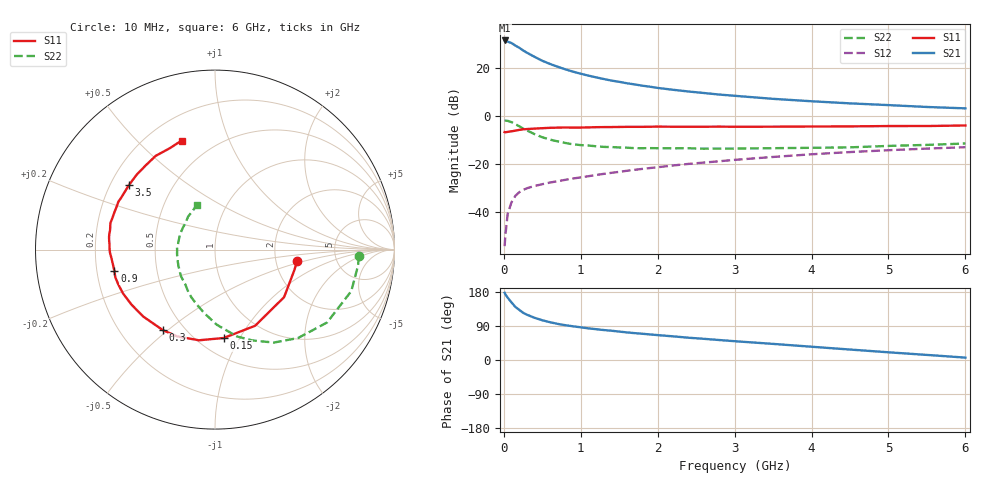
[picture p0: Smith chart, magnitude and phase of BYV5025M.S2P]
! SIEMENS Small Signal Semiconductors
! BFY420
! Si NPN RF SIEGET Grounded Emitter Transistor in MICRO-X
! VCE = 0.5 V  IC = 25 mA
! Common Emitter S-Parameters:  October  1996
# GHz  S  MA  R  50
!  f  S11  S21  S12  S22
! GHz  MAG  ANG  MAG  ANG  MAG  ANG  MAG  ANG
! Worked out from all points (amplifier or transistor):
!   36 points, 10 MHz to 6 GHz, reference 50 ohm
!   highest |S21| = 31.6 dB at 10 MHz (marker M1)
!   |S21| within 3 dB of that: start of sweep to 197 MHz
!   unconditionally stable (mu >= 1): start of sweep to 23.53 MHz; 1.099 GHz to end of sweep
!   at 250 MHz: K = 0.42, MSG = 29.2 dB, |S12| = -30.9 dB
!   at 1.4 GHz: K = 1.08, MAG = 17.6 dB, |S12| = -23.7 dB
!   at 6 GHz: K = 1.18, MAG = 5.6 dB, |S12| = -13.0 dB
!   S11 on the Smith chart (normalised r, x): 10 MHz: 2.64, -0.43; 150 MHz: 0.66, -0.86; 300 MHz: 0.38, -0.48; 900 MHz: 0.27, -0.10; 3.5 GHz: 0.28, +0.31; 6 GHz: 0.34, +0.68
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0.01  0.4621 -7.9  38.1 177.4  0.0019 97.3  0.8015 -2.6
0.02  0.4564 -14.8  37.83 173.2  0.0032 85.3  0.8022 -6.2
0.05  0.4673 -34.5  36.03 164.4  0.009 79.1  0.7939 -16.9
0.1  0.4796 -62.2  33.61 151.9  0.0158 69.6  0.745 -33.0
0.15  0.4949 -84.4  29.78 140.1  0.0215 60.8  0.6758 -46.8
0.2  0.5132 -100.1  26.81 132.4  0.0255 56.7  0.6128 -57.7
0.25  0.5273 -113.5  23.61 124.7  0.0285 51.8  0.5469 -67.7
0.3  0.5345 -122.9  21.12 119.5  0.0309 49.4  0.4992 -75.8
0.4  0.5466 -136.9  17.29 111.3  0.0345 47.5  0.4183 -88.7
0.5  0.5571 -146.6  14.32 104.9  0.0376 46.7  0.3602 -99.3
0.6  0.5674 -154.3  12.29 99.7  0.0407 46.1  0.3215 -108.6
0.7  0.5724 -159.9  10.75 95.3  0.0434 47.2  0.2952 -116.9
0.9  0.5733 -167.8  8.476 88.9  0.0494 47.7  0.2561 -129.9
1.1  0.5793 -175.5  7.006 83.5  0.0552 49.0  0.2415 -141.2
1.3  0.5875 179.5  5.947 79.0  0.0618 49.6  0.2264 -151.0
1.6  0.5947 173.1  4.849 72.8  0.0717 49.6  0.2181 -162.2
2.2  0.5981 162.9  3.543 62.4  0.0925 48.0  0.2112 -178.7
2.8  0.6008 153.6  2.816 52.7  0.1134 44.7  0.2087 168.0
3.5  0.5994 143.2  2.29 42.5  0.1395 39.6  0.2128 156.2
4.5  0.6078 129.2  1.842 27.6  0.1765 29.7  0.2215 137.5
5.5  0.6185 114.0  1.548 13.4  0.2087 18.8  0.2493 119.8
6  0.6354 107.0  1.448 6.3  0.2232 13.5  0.2667 112.7
